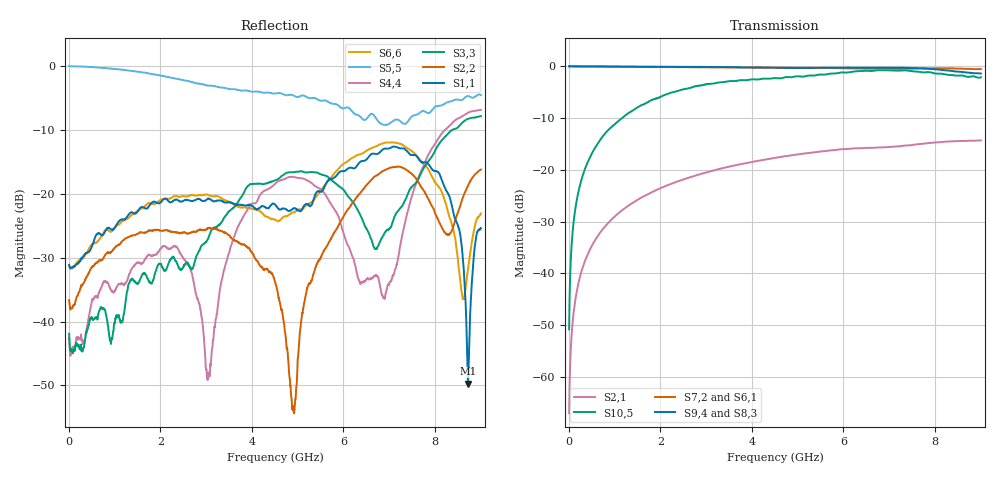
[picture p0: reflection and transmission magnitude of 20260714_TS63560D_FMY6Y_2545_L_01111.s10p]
# GHz S DB R 50
! CMT, SN0916, 25263762, 26.7.0
! Date: 15.07.2026 13:40:53
! Data: Format
! Freq S1.1:dB/Ang S1.2:dB/Ang S1.3:dB/Ang S1.4:dB/Ang S1.5:dB/Ang S1.6:dB/Ang S1.7:dB/Ang S1.8:dB/Ang S1.9:dB/Ang S1.10:dB/Ang
!  S2.1:dB/Ang S2.2:dB/Ang S2.3:dB/Ang S2.4:dB/Ang S2.5:dB/Ang S2.6:dB/Ang S2.7:dB/Ang S2.8:dB/Ang S2.9:dB/Ang S2.10:dB/Ang
!  S3.1:dB/Ang S3.2:dB/Ang S3.3:dB/Ang S3.4:dB/Ang S3.5:dB/Ang S3.6:dB/Ang S3.7:dB/Ang S3.8:dB/Ang S3.9:dB/Ang S3.10:dB/Ang
!  S4.1:dB/Ang S4.2:dB/Ang S4.3:dB/Ang S4.4:dB/Ang S4.5:dB/Ang S4.6:dB/Ang S4.7:dB/Ang S4.8:dB/Ang S4.9:dB/Ang S4.10:dB/Ang
!  S5.1:dB/Ang S5.2:dB/Ang S5.3:dB/Ang S5.4:dB/Ang S5.5:dB/Ang S5.6:dB/Ang S5.7:dB/Ang S5.8:dB/Ang S5.9:dB/Ang S5.10:dB/Ang
!  S6.1:dB/Ang S6.2:dB/Ang S6.3:dB/Ang S6.4:dB/Ang S6.5:dB/Ang S6.6:dB/Ang S6.7:dB/Ang S6.8:dB/Ang S6.9:dB/Ang S6.10:dB/Ang
!  S7.1:dB/Ang S7.2:dB/Ang S7.3:dB/Ang S7.4:dB/Ang S7.5:dB/Ang S7.6:dB/Ang S7.7:dB/Ang S7.8:dB/Ang S7.9:dB/Ang S7.10:dB/Ang
!  S8.1:dB/Ang S8.2:dB/Ang S8.3:dB/Ang S8.4:dB/Ang S8.5:dB/Ang S8.6:dB/Ang S8.7:dB/Ang S8.8:dB/Ang S8.9:dB/Ang S8.10:dB/Ang
!  S9.1:dB/Ang S9.2:dB/Ang S9.3:dB/Ang S9.4:dB/Ang S9.5:dB/Ang S9.6:dB/Ang S9.7:dB/Ang S9.8:dB/Ang S9.9:dB/Ang S9.10:dB/Ang
!  S10.1:dB/Ang S10.2:dB/Ang S10.3:dB/Ang S10.4:dB/Ang S10.5:dB/Ang S10.6:dB/Ang S10.7:dB/Ang S10.8:dB/Ang S10.9:dB/Ang S10.10:dB/Ang
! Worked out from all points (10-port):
!   2001 points, 10 MHz to 9 GHz, reference 50 ohm
!   strongest paths, dB at 10 MHz, 2.257 GHz, 4.505 GHz, 6.753 GHz, 9 GHz:
!     S9,4: -0.1, -0.2, -0.4, -0.4, -1.5
!     S7,2: -0.1, -0.3, -0.4, -0.6, -0.6
!     S8,3: -0.1, -0.2, -0.4, -0.4, -1.3
!     S6,1: -0.3, -0.4, -0.5, -0.7, -0.6
!     S10,5: -50.8, -5.1, -2.4, -0.8, -2.2
!     S2,1: -66.9, -22.7, -17.7, -15.7, -14.4
!   lowest |S11| = -49.7 dB at 8.721 GHz (marker M1), VSWR 1.01, Z = 49.9 + j0.297 ohm
!   |S11| at or under -10 dB: start of sweep to end of sweep
